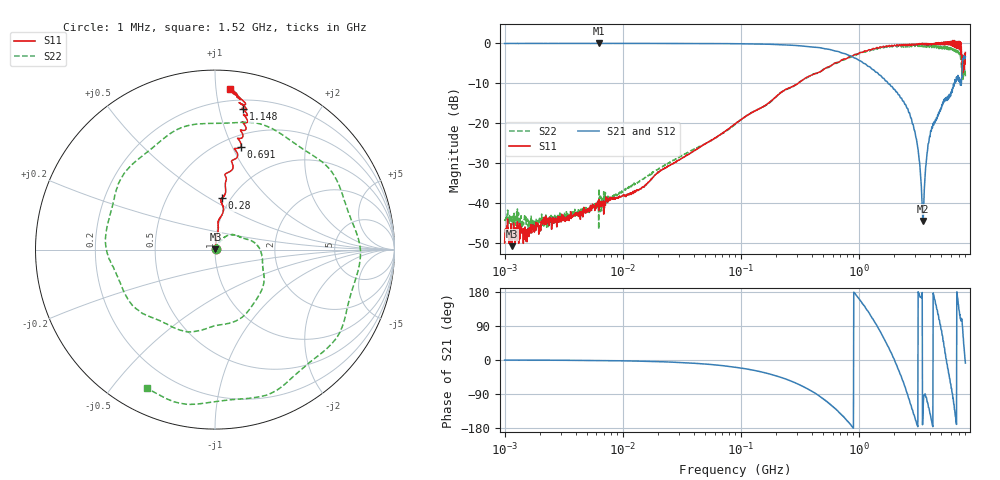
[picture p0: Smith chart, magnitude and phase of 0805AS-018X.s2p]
!s-Parameter Generated by FASTRON Sdn. Bhd.
!FASTRON P/N : 0805AS-018X
!Keysight Technologies: E5071C_MY46733604_B.14.02
!Date: Mon Jun 15 12:49:22 2026
!Version  :Rev01  Mon Jun 15 12:49:22 2026
!Data & Calibration Information:
!Freq  S11:SOLT2(ON)  S21:SOLT2(ON)  S12:SOLT2(ON)  S22:SOLT2(ON)
!PortZ  Port1:50+j0  Port2:50+j0
!When reading reference impedance value at option line is always used.
! Remarks : This data is being provided solely for informational purposes.
# Hz S dB R 50
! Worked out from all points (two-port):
!   1601 points, 1 MHz to 8 GHz, reference 50 ohm
!   highest |S21| = -0.02 dB at 6.301 MHz (marker M1); lowest = -44.4 dB at 3.508 GHz (marker M2)
!   |S21| within 3 dB of the highest: start of sweep to 817.3 MHz
!   lowest |S11| = -50.7 dB at 1.152 MHz (marker M3), VSWR 1.01, Z = 50.3 + j0.0911 ohm
!   |S11| at or under -10 dB: start of sweep to 306.4 MHz
!   |S22| runs from -46.5 to -0.4 dB; largest |S21 - S12| = 0.013
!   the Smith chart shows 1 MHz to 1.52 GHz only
!   S11 on the Smith chart (normalised r, x): 1 MHz: 1.01, +0.00; 280 MHz: 0.91, +0.58; 691 MHz: 0.61, +1.08; 1.148 GHz: 0.27, +1.18; 1.52 GHz: 0.12, +1.09
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1000000  -49.90 15.7  -0.07 -0.3  -0.04 -0.2  -44.40 10.5
1151819  -50.70 18.1  -0.07 -0.3  -0.04 -0.2  -43.40 13.4
4479405  -42.90 46.2  -0.06 -1.0  -0.05 -1.0  -42.50 46.2
6301378  -39.00 51.3  -0.02 -1.5  -0.02 -1.4  -36.30 48.4
2.00676e7  -32.20 76.8  -0.07 -4.3  -0.07 -4.3  -31.40 65.1
8.994653e7  -20.10 80.7  -0.14 -19.1  -0.14 -19.1  -20.30 50.1
2.800228e8  -10.70 82.1  -0.54 -58.3  -0.53 -58.2  -10.80 -22.4
4.006501e8  -7.92 81.0  -0.96 -82.5  -0.95 -82.5  -7.83 -68.0
6.909832e8  -4.59 76.0  -2.24 -140.0  -2.23 -140.0  -4.49 -177.0
1.14826e9  -1.94 78.6  -5.27 136.0  -5.26 136.0  -2.19 12.3
1.519696e9  -0.91 84.6  -8.01 75.3  -8.02 75.2  -1.30 -116.0
1.7949e9  -0.65 92.0  -10.20 32.7  -10.20 32.5  -0.86 151.0
2.189041e9  -0.45 106.0  -12.90 -27.8  -12.90 -28.1  -0.84 15.3
2.501569e9  -0.28 115.0  -15.40 -77.0  -15.40 -77.2  -0.99 -94.2
3.015098e9  -0.34 123.0  -22.90 -157.0  -22.90 -157.0  -0.58 91.9
3.507506e9  -0.18 148.0  -44.40 -129.0  -44.40 -129.0  -0.53 -75.1
4.075033e9  -0.20 155.0  -21.80 -152.0  -21.80 -153.0  -0.98 87.9
4.57657e9  -0.13 174.0  -18.60 134.0  -18.70 134.0  -0.77 -81.8
5.164399e9  0.06 -155.0  -14.70 52.3  -14.80 52.4  -0.98 83.5
5.668252e9  -0.33 -146.0  -13.90 -23.2  -13.90 -23.0  -0.94 -76.5
6.226476e9  0.67 -90.9  -11.20 -89.4  -11.20 -89.8  -1.79 93.5
8e9  -2.32 -39.3  -3.39 -8.1  -3.25 -7.8  -8.34 -137.0
